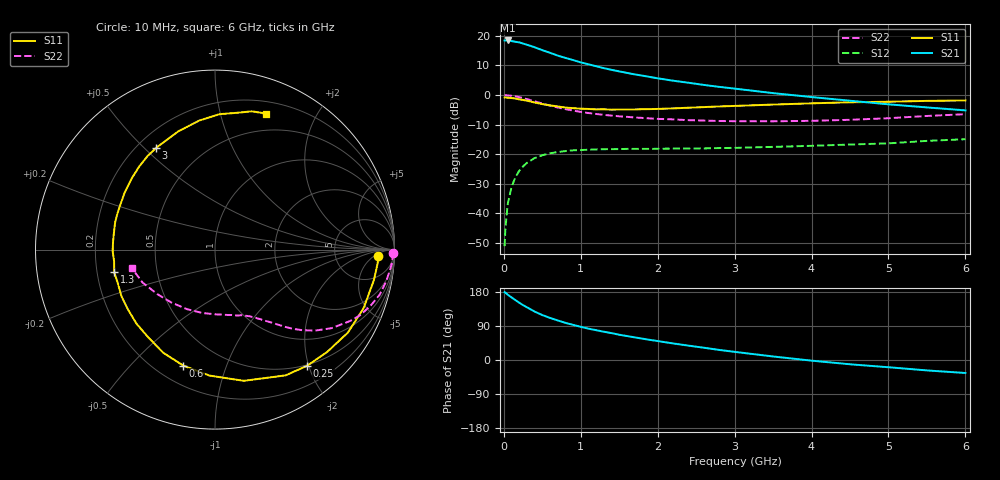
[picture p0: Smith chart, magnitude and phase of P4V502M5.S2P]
! SIEMENS Small Signal Semiconductors
! BFP182
! Si NPN RF Bipolar Junction Transistor in SOT143
! VCE = 0.5 V  IC = 2.5 mA
! Common Emitter S-Parameters:  March  1996
# GHz  S  MA  R  50
!  f  S11  S21  S12  S22
! GHz  MAG  ANG  MAG  ANG  MAG  ANG  MAG  ANG
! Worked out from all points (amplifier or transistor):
!   36 points, 10 MHz to 6 GHz, reference 50 ohm
!   highest |S21| = 18.4 dB at 50 MHz (marker M1)
!   |S21| within 3 dB of that: start of sweep to 471.7 MHz
!   unconditionally stable (mu >= 1): 1.827 GHz to end of sweep
!   at 250 MHz: K = 0.16, MSG = 20.7 dB, |S12| = -24.1 dB
!   at 1.4 GHz: K = 0.81, MSG = 13.4 dB, |S12| = -18.3 dB
!   at 6 GHz: K = 1.24, MAG = 1.9 dB, |S12| = -14.9 dB
!   S11 on the Smith chart (normalised r, x): 10 MHz: 18, -7; 250 MHz: 0.48, -1.97; 600 MHz: 0.31, -0.72; 1.3 GHz: 0.27, -0.10; 3 GHz: 0.27, +0.54; 6 GHz: 0.32, +1.40
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0.01  0.9072 -2.2  8.335 178.9  0.0028 88.6  0.9902 -1.0
0.02  0.91 -4.5  8.358 177.6  0.0055 86.9  0.9915 -2.1
0.05  0.9014 -10.9  8.362 172.5  0.0143 84.0  0.9864 -5.2
0.15  0.8728 -32.0  7.94 158.1  0.0408 71.4  0.9514 -15.3
0.2  0.8459 -42.4  7.768 151.1  0.0525 66.1  0.9216 -19.8
0.25  0.8259 -51.6  7.404 144.7  0.0625 60.8  0.8883 -24.2
0.3  0.8036 -60.7  7.085 139.2  0.0716 56.3  0.8533 -27.7
0.4  0.7485 -77.6  6.419 127.8  0.0861 48.1  0.7841 -33.9
0.5  0.7027 -92.5  5.734 118.6  0.0961 41.1  0.7185 -38.9
0.6  0.6699 -105.3  5.177 111.1  0.1038 35.9  0.6623 -42.7
0.7  0.6432 -116.5  4.642 104.4  0.109 31.6  0.6171 -45.6
0.8  0.6144 -127.2  4.245 98.1  0.113 28.1  0.5792 -47.9
0.9  0.6014 -136.6  3.901 92.7  0.1164 25.1  0.5471 -49.9
1.1  0.5824 -153.7  3.308 82.7  0.1195 20.3  0.4967 -53.7
1.3  0.5757 -167.3  2.849 74.6  0.1216 16.7  0.4627 -56.9
1.7  0.5713 169.7  2.235 59.8  0.1232 12.5  0.4178 -62.7
2.2  0.5956 147.6  1.748 43.7  0.1246 9.9  0.3882 -71.2
3  0.655 120.1  1.285 21.5  0.1281 8.0  0.3614 -88.6
3.5  0.6904 107.1  1.078 9.3  0.1332 7.5  0.3601 -101.3
4.5  0.7549 88.1  0.802 -11.3  0.146 6.5  0.3821 -129.5
5.5  0.7971 75.1  0.618 -27.5  0.1682 4.8  0.4433 -155.5
6  0.8101 69.3  0.551 -34.3  0.1793 1.8  0.475 -167.5
